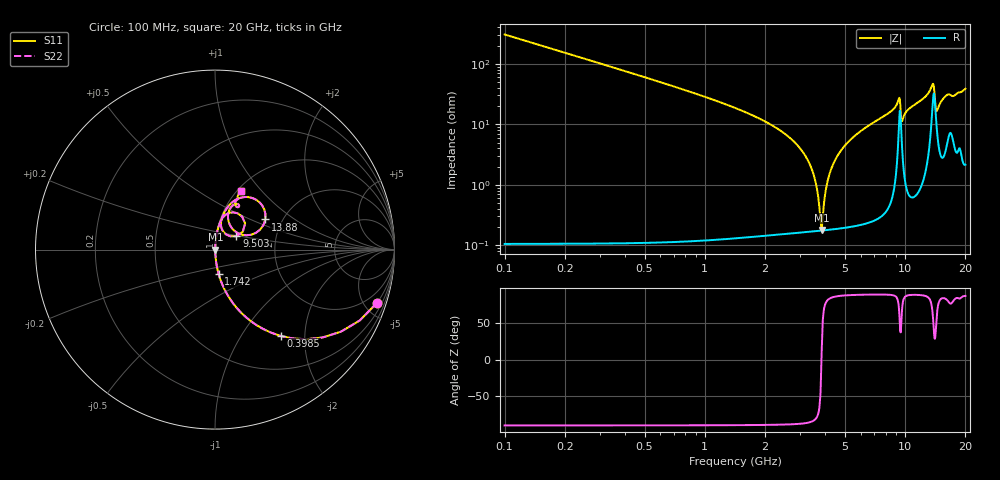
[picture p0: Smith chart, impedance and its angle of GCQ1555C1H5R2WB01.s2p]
!Murata Part Number: GCQ1555C1H5R2WB01
!These Parameters are Measured in Series Mode Connection
!Data Generated on Jan 08, 2026
!  o--ll--o
!Port1  Port2
!  o------o
!Operation Temp=25[degC], DC Bias Voltage=0[V]
!Freq. Start=100[MHz] Stop=20[GHz] 401[Steps]
# Hz S RI R 50
!Freq.(Hz) S11(Real) S11(Imag) S21(Real) S21(Imag) S12(Real) S12(Imag) S22(Real) S22(Imag)
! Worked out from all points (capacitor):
!   401 points, 100 MHz to 20 GHz, reference 50 ohm
!   read as one part in series: C = 5.2 pF near 199.5 MHz
!   lowest |Z| = 178 mohm at 3.831 GHz (marker M1)
!   series resonance near 3.823 GHz, so ESL is about 330 pH
!   S11 on the Smith chart (normalised r, x): 100 MHz: 1.00, -6.12; 398.5 MHz: 1.00, -1.52; 1.742 GHz: 1.00, -0.28; 9.503 GHz: 1.25, +0.19; 13.88 GHz: 1.64, +0.61; 20 GHz: 1.04, +0.77
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1e8  0.9033 -0.2953  0.0967 0.2953  0.0967 0.2953  0.9033 -0.2953
3.985e8  0.3661 -0.481  0.6339 0.481  0.6339 0.481  0.3661 -0.481
8.4625e8  0.1066 -0.3069  0.8934 0.3069  0.8934 0.3069  0.1066 -0.3069
1.74175e9  0.0204 -0.1363  0.9796 0.1363  0.9796 0.1363  0.0204 -0.1363
2.83625e9  0.00395 -0.0485  0.9961 0.0485  0.9961 0.0485  0.00395 -0.0485
3.43325e9  0.00198 -0.0173  0.998 0.0173  0.998 0.0173  0.00198 -0.0173
3.73175e9  0.00175 -0.0039  0.9983 0.0039  0.9983 0.0039  0.00175 -0.0039
3.83125e9  0.00175 0.000332  0.9983 -0.000332  0.9983 -0.000332  0.00175 0.000332
4.1795e9  0.00201 0.0144  0.998 -0.0144  0.998 -0.0144  0.00201 0.0144
4.62725e9  0.00284 0.0311  0.9972 -0.0311  0.9972 -0.0311  0.00284 0.0311
5.473e9  0.00562 0.0597  0.9944 -0.0597  0.9944 -0.0597  0.00562 0.0597
6.7665e9  0.0125 0.0998  0.9875 -0.0998  0.9875 -0.0998  0.0125 0.0998
9.30375e9  0.1242 0.2029  0.8758 -0.2029  0.8758 -0.2029  0.1242 0.2029
9.50275e9  0.1194 0.075  0.8806 -0.075  0.8806 -0.075  0.1194 0.075
9.652e9  0.0501 0.0953  0.9499 -0.0953  0.9499 -0.0953  0.0501 0.0953
1.005e10  0.033 0.1487  0.967 -0.1487  0.967 -0.1487  0.033 0.1487
1.338325e10  0.1639 0.2926  0.8361 -0.2926  0.8361 -0.2926  0.1639 0.2926
1.388075e10  0.2803 0.1678  0.7197 -0.1678  0.7197 -0.1678  0.2803 0.1678
1.43285e10  0.1058 0.1071  0.8942 -0.1071  0.8942 -0.1071  0.1058 0.1071
1.547275e10  0.0868 0.2325  0.9132 -0.2325  0.9132 -0.2325  0.0868 0.2325
1.67165e10  0.1348 0.2437  0.8652 -0.2437  0.8652 -0.2437  0.1348 0.2437
2e10  0.1437 0.3241  0.8563 -0.3241  0.8563 -0.3241  0.1437 0.3241
